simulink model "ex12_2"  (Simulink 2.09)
settings: Solver=ode113  StartTime=0.0  StopTime=500  FixedStep=.1  RelTol=1e-3  AbsTol=1e-6
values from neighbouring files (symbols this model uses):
  K11 = 1/((m1+m2)*r1^2)    (= 0.0166666666667)    [ex12_2st.m]
  K12 = m2*r1*r2    (= 15)    [ex12_2st.m]
  K21 = K12    (= 15)    [ex12_2st.m]
  K22 = 1/(m2*r2^2)    (= 0.0888888888889)    [ex12_2st.m]

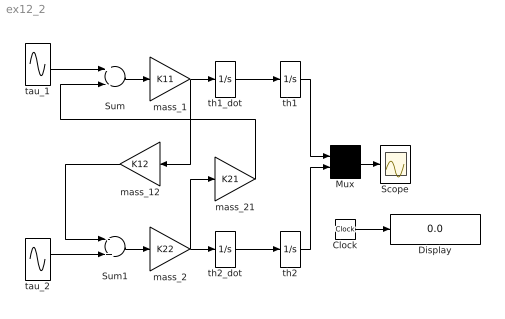
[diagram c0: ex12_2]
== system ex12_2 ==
  Clock : Clock
  Display : Display
  Mux : Mux  Inputs=2
  Scope : Scope
  Sum : Sum  Inputs=+-
  Sum1 : Sum  Inputs=-+
  mass_1 : Gain  Gain=K11
  mass_12 : Gain  Orientation=left  Gain=K12
  mass_2 : Gain  Gain=K22
  mass_21 : Gain  Gain=K21
  tau_1 : Sin  Amplitude=1  Frequency=0.1  Phase=0  SampleTime=-1
  tau_2 : Sin  Amplitude=1  Frequency=0.2  Phase=-1  SampleTime=-1
  th1 : Integrator  ExternalReset=none  InitialConditionSource=internal  InitialCondition=0  LimitOutput=off  UpperSaturationLimit=inf  LowerSaturationLimit=-inf  ShowSaturationPort=off  ShowStatePort=off  AbsoluteTolerance=auto
  th1_dot : Integrator  ExternalReset=none  InitialConditionSource=internal  InitialCondition=0  LimitOutput=off  UpperSaturationLimit=inf  LowerSaturationLimit=-inf  ShowSaturationPort=off  ShowStatePort=off  AbsoluteTolerance=auto
  th2 : Integrator  ExternalReset=none  InitialConditionSource=internal  InitialCondition=0  LimitOutput=off  UpperSaturationLimit=inf  LowerSaturationLimit=-inf  ShowSaturationPort=off  ShowStatePort=off  AbsoluteTolerance=auto
  th2_dot : Integrator  ExternalReset=none  InitialConditionSource=internal  InitialCondition=0  LimitOutput=off  UpperSaturationLimit=inf  LowerSaturationLimit=-inf  ShowSaturationPort=off  ShowStatePort=off  AbsoluteTolerance=auto
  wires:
  Clock/1 -> Display/1
  Mux/1 -> Scope/1
  th2/1 -> Mux/2
  th1/1 -> Mux/1
  mass_1/1 -> mass_12/1, th1_dot/1
  mass_21/1 -> Sum/2
  mass_12/1 -> Sum1/1
  tau_2/1 -> Sum1/2
  tau_1/1 -> Sum/1
  mass_2/1 -> mass_21/1, th2_dot/1
  Sum1/1 -> mass_2/1
  Sum/1 -> mass_1/1
  th2_dot/1 -> th2/1
  th1_dot/1 -> th1/1
